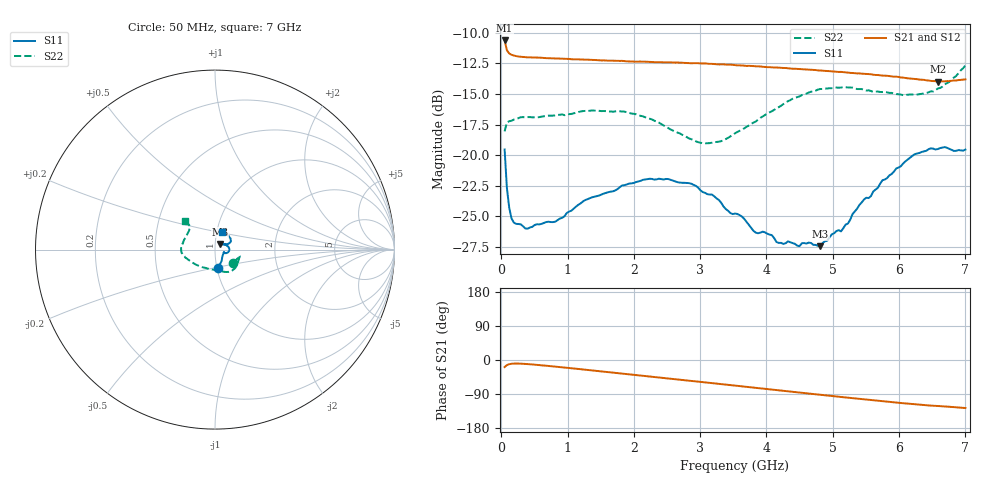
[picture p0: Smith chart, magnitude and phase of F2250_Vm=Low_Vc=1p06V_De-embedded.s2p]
! Integrated Device Technology
! Corporate Headquarters
! 6024 Silver Creek Valley Road
! San Jose, CA 95138  USA
! Phone:  1-408-284-8200
! Toll Free:  1-800-223-1366
! Webpage:  http://www.idt.com/
! Timing and RF Division
! 515 Groton Road, Suite 102
! Westford, MA 01886-6024
! Device:  F2250
! Description: Voltage Variable RF Attenuator
! Frequency:  50.0 -  6000.00 MHz
! Package:  3x3 mm Thin QFN Plastic Package: 16 pin
! Ports:  2 RF, 3 DC
!  Pin  1  = GND
!  Pin  2  = NC
!  Pin  3  = RF1  = Port 1
!  Pin  4  = NC
!  Pin  5  = GND
!  Pin  6  = GND
!  Pin  7  = GND
!  Pin  8  = GND
!  Pin  9  = NC
!  Pin 10  = RF2  = Port 2
!  Pin 11  = NC
!  Pin 12  = GND
!  Pin 13  = GND
!  Pin 14  = VCNTRL
!  Pin 15  = VDD
!  Pin 16  = VMODE
! Vcntrl:  1.060 Volts
! Vmode:  +0.000 Volts
! Vdd:  +3.30  Volts
! Current:  1.190 mA
! Data:  The device was measured on a the F2250 evaluation board which has
!  individual transmission lines to the RF pins.  Data was collected
!  using a calibrated network analyzer.  The evaluation board was
!  de-embedded using a TRL calibration technique.
!  The reference plane is the edge of the package pin.
! Misc:  SN 10
!  Action Tracker AT0258
! Date Measured:  2014-11-26
! Date:  2015-10-15  MJV
! Note:
!  Integrated Device Technology supplies this data as a sample of measured
!  data at the package pin for this product.  Your particular data for this
!  product may vary.
!  Data was taken at 25 degrees C.
!  Integrated Device Technology reserves the right to change this data at anytime.
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# GHz S dB R 50
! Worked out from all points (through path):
!   201 points, 50 MHz to 7 GHz, reference 50 ohm
!   highest |S21| = -10.62 dB at 50 MHz (marker M1); lowest = -14.0 dB at 6.583 GHz (marker M2)
!   group delay of S21, straight-line fit = 50.2 ps
!   lowest |S11| = -27.4 dB at 4.811 GHz (marker M3), VSWR 1.09, Z = 52.8 + j3.34 ohm
!   |S11| at or under -10 dB: start of sweep to end of sweep
!   |S22| runs from -19.0 to -12.7 dB; largest |S21 - S12| = 0.00071
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0.05  -19.53 -80.6  -10.62 -18.6  -10.61 -18.6  -18.05 -36.0
0.08475  -22.69 -59.9  -11.42 -13.4  -11.41 -13.4  -17.31 -20.1
0.1195  -24.30 -48.9  -11.68 -11.1  -11.67 -11.0  -17.23 -15.4
0.189  -25.51 -34.4  -11.85 -9.5  -11.85 -9.5  -17.09 -13.5
0.3975  -26.01 -20.2  -12.00 -10.8  -11.99 -10.8  -16.89 -15.9
0.8145  -25.44 -16.9  -12.10 -17.5  -12.09 -17.5  -16.74 -28.8
1.2315  -23.78 -17.4  -12.18 -24.9  -12.18 -24.9  -16.39 -40.2
1.857  -22.45 -10.0  -12.30 -36.2  -12.31 -36.2  -16.44 -53.4
2.37825  -21.92 -0.6  -12.39 -45.8  -12.39 -45.8  -17.34 -66.2
2.86475  -22.33 11.9  -12.48 -55.0  -12.47 -55.0  -18.69 -87.1
3.0385  -23.01 16.6  -12.50 -58.3  -12.48 -58.3  -19.03 -97.5
3.525  -24.78 31.8  -12.63 -67.5  -12.64 -67.6  -18.21 -128.3
3.83775  -26.33 44.0  -12.73 -73.4  -12.72 -73.4  -17.25 -144.1
4.18525  -27.17 53.6  -12.84 -80.0  -12.84 -80.0  -16.07 -158.3
4.7065  -27.33 52.8  -13.02 -89.8  -13.01 -89.8  -14.78 -172.0
4.81075  -27.44 48.0  -13.07 -91.7  -13.07 -91.7  -14.59 -173.9
5.1235  -26.23 38.0  -13.19 -97.5  -13.17 -97.6  -14.47 178.9
5.471  -23.62 28.0  -13.34 -103.8  -13.34 -103.8  -14.68 171.4
5.85325  -21.65 23.5  -13.53 -110.6  -13.53 -110.6  -14.91 161.3
6.2355  -19.92 28.2  -13.77 -116.9  -13.76 -117.0  -15.05 148.7
6.583  -19.50 40.1  -13.98 -121.5  -13.97 -121.5  -14.55 138.7
7  -19.54 68.8  -13.80 -126.7  -13.81 -126.8  -12.66 136.7
